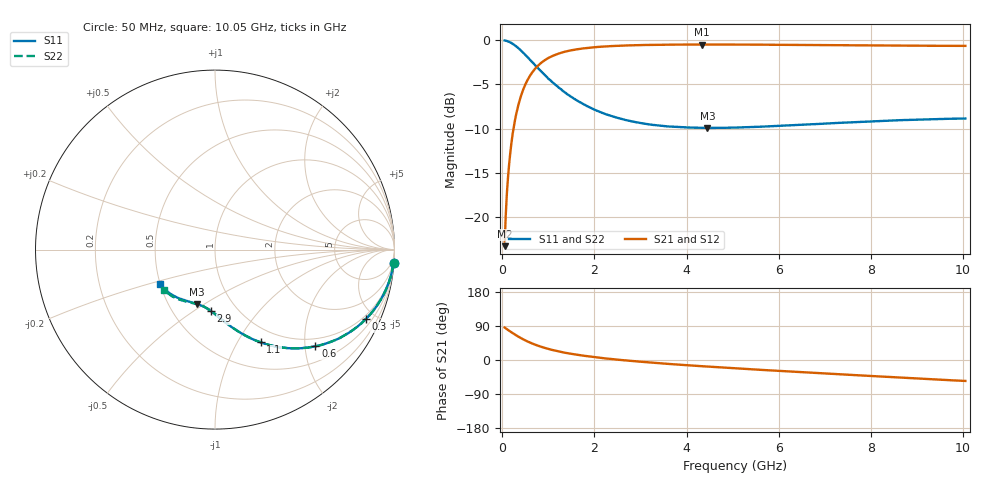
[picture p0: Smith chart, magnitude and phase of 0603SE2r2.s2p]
! AVX Thin Film Operation		Date: August 2001
! Description: Accu-P® Series, Thin Film, SMD, RF Capacitor
! Part Number: 06035J2R2ABT
! 50 MHz  -  10.05 GHz
! Serial Measurements
# mhz S db R 50
!	S11		S21		S12		S22
!	dB	Phase	dB	Phase	dB	Phase	dB	Phase
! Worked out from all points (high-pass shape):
!   401 points, 50 MHz to 10.05 GHz, reference 50 ohm
!   highest |S21| = -0.48 dB at 4.325 GHz (marker M1); lowest = -23.3 dB at 50 MHz (marker M2)
!   |S21| within 3 dB of the highest: 672.1 MHz to end of sweep
!   lowest |S11| = -9.9 dB at 4.45 GHz (marker M3), VSWR 1.94, Z = 34.6 - j23.4 ohm
!   |S11| at or under -10 dB: nowhere
!   |S22| runs from -9.9 to 0.0 dB; largest |S21 - S12| = 0
!   S11 on the Smith chart (normalised r, x): 50 MHz: 1, -26; 300 MHz: 0.82, -4.40; 600 MHz: 0.82, -2.23; 1.1 GHz: 0.81, -1.25; 2.9 GHz: 0.76, -0.59; 10.05 GHz: 0.50, -0.22
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50  -0.02 -4.3  -23.30 85.7  -23.30 85.7  -0.02 -4.3
75  -0.05 -6.5  -19.76 83.4  -19.76 83.4  -0.05 -6.5
125  -0.13 -10.8  -15.42 79.2  -15.42 79.2  -0.13 -10.8
175  -0.24 -14.9  -12.65 75.1  -12.65 75.1  -0.24 -14.9
225  -0.40 -19.0  -10.57 71.0  -10.57 71.0  -0.40 -19.0
300  -0.68 -24.8  -8.39 65.2  -8.39 65.2  -0.68 -24.8
425  -1.26 -33.5  -6.00 56.4  -6.00 56.4  -1.26 -33.5
600  -2.20 -43.9  -4.02 46.0  -4.02 46.0  -2.20 -43.9
725  -2.89 -50.1  -3.14 39.9  -3.14 39.9  -2.89 -50.1
850  -3.56 -55.3  -2.53 34.7  -2.53 34.7  -3.56 -55.3
1100  -4.80 -63.9  -1.75 26.1  -1.75 26.1  -4.80 -63.9
1375  -5.95 -71.0  -1.27 19.0  -1.27 19.0  -5.95 -70.9
1725  -7.12 -78.0  -0.94 12.0  -0.94 12.0  -7.12 -77.8
2225  -8.33 -85.7  -0.70 4.3  -0.70 4.3  -8.32 -85.4
2900  -9.27 -93.7  -0.56 -3.5  -0.56 -3.5  -9.26 -93.0
3400  -9.65 -98.7  -0.51 -8.5  -0.51 -8.5  -9.65 -97.9
4325  -9.91 -107.0  -0.48 -16.3  -0.48 -16.3  -9.90 -105.5
4450  -9.92 -108.0  -0.48 -17.3  -0.48 -17.3  -9.90 -106.3
5050  -9.88 -113.0  -0.49 -21.9  -0.49 -21.9  -9.86 -111.0
6725  -9.51 -125.0  -0.54 -33.7  -0.54 -33.7  -9.48 -122.0
8400  -9.09 -137.1  -0.60 -44.8  -0.60 -44.8  -9.06 -132.1
10050  -8.85 -147.8  -0.63 -55.2  -0.63 -55.2  -8.82 -141.8
